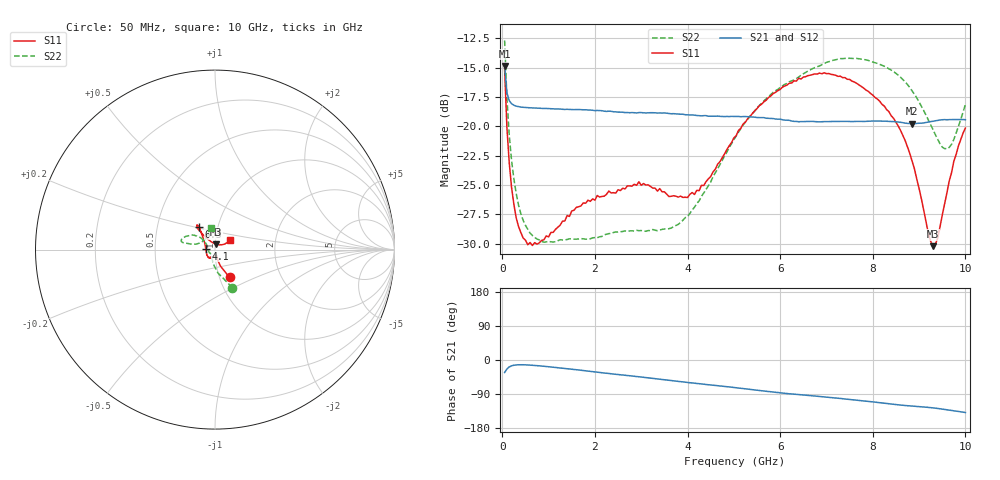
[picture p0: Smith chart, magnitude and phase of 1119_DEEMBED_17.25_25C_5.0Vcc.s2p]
!Hittite Microwave Corp.
!Digital Attenuator/PhaseShifter Rev 1.4.0
!Filename: C:\DATA\DATA\1119_DEEMBED_17.25_25C_5.0Vcc.s2p
!VNA ID: Agilent Technologies,N5224A,MY51441122,A.10.45.03
!Device type:
!2 Port Calibration.
!Temp(C): 25
!Lot Number:
!Serial Number:
!Operator:
!Misc:
!Attenuator:  17.250
# GHZ S DB R 50.0
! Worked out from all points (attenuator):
!   200 points, 50 MHz to 10 GHz, reference 50 ohm
!   highest |S21| = -14.85 dB at 50 MHz (marker M1); lowest = -19.8 dB at 8.85 GHz (marker M2)
!   lowest |S11| = -30.2 dB at 9.3 GHz (marker M3), VSWR 1.06, Z = 50.6 + j3.04 ohm
!   |S11| at or under -10 dB: start of sweep to end of sweep
!   |S22| runs from -29.9 to -12.7 dB; largest |S21 - S12| = 0.0005
!   S11 on the Smith chart (normalised r, x): 50 MHz: 1.12, -0.36; 4.1 GHz: 0.90, +0.01; 6.3 GHz: 0.81, +0.21; 10 GHz: 1.17, +0.13
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0.05  -15.13 -62.4  -14.85 -33.0  -14.86 -33.1  -12.68 -65.4
0.1  -20.14 -71.4  -17.16 -23.7  -17.16 -23.6  -17.62 -82.8
0.2  -25.21 -74.9  -18.07 -15.4  -18.07 -15.4  -22.90 -99.5
0.3  -27.80 -75.2  -18.28 -13.0  -18.28 -13.0  -25.71 -109.4
0.45  -29.52 -75.4  -18.38 -12.6  -18.38 -12.6  -28.01 -119.9
0.85  -29.73 -86.7  -18.47 -15.9  -18.47 -16.0  -29.82 -132.9
1.75  -26.53 -110.8  -18.59 -27.8  -18.59 -27.9  -29.59 -138.3
2.95  -24.73 -130.7  -18.83 -44.1  -18.84 -44.2  -28.90 -157.3
3.4  -25.31 -148.1  -18.86 -50.6  -18.87 -50.7  -28.84 -170.6
4.1  -25.65 174.1  -19.03 -60.7  -19.03 -60.7  -27.14 161.2
4.35  -25.05 160.6  -19.09 -63.8  -19.10 -63.9  -25.69 151.7
5.05  -20.80 135.8  -19.16 -73.2  -19.18 -73.2  -20.83 140.4
5.65  -17.91 128.0  -19.26 -81.8  -19.27 -81.9  -17.83 143.6
6.3  -16.12 125.3  -19.58 -90.1  -19.59 -90.2  -16.04 149.5
6.7  -15.59 126.5  -19.58 -94.4  -19.60 -94.4  -15.08 154.9
7.5  -16.00 129.1  -19.59 -104.2  -19.59 -104.2  -14.20 163.9
8.35  -18.76 128.9  -19.58 -115.5  -19.58 -115.5  -15.09 167.6
8.85  -22.99 124.0  -19.77 -121.5  -19.77 -121.5  -16.98 167.0
9.3  -30.22 76.3  -19.57 -126.3  -19.58 -126.4  -20.27 158.8
9.400001  -29.55 55.6  -19.50 -127.8  -19.51 -127.8  -21.10 152.5
9.65  -24.67 30.8  -19.43 -132.2  -19.44 -132.2  -21.80 126.6
10  -20.15 33.2  -19.44 -138.5  -19.44 -138.5  -18.13 99.5
